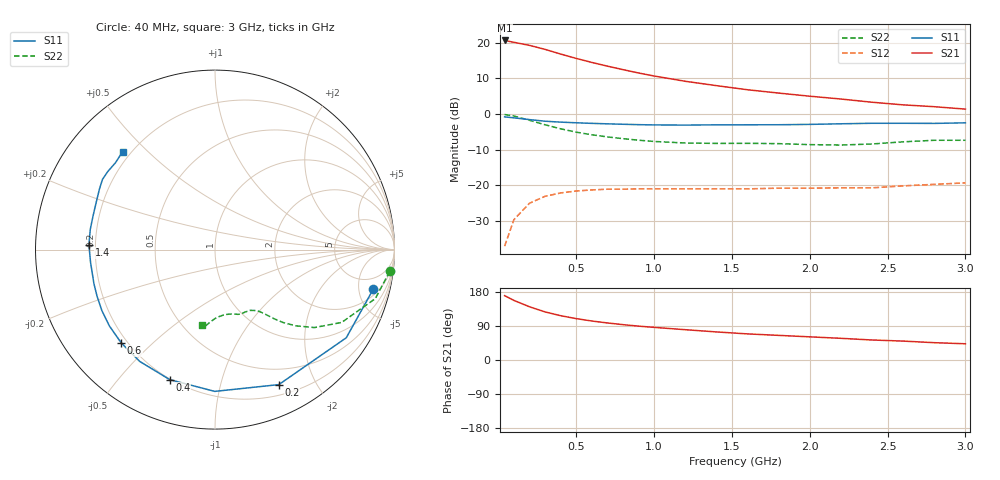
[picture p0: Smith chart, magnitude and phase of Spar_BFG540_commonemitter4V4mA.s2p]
! Filename:  BFG540A.S2P  Version:  3.0
! NXP part #: BFG540  Date: Feb 1992
! Bias condition: Vce=4V, Ic=4mA
! IN LINE PINNING: same data as with cross emitter pinning.
#  MHz  S  MA  R  50
! Freq  S11  S21  S12  S22  !GUM [dB]
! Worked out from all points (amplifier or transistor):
!   21 points, 40 MHz to 3 GHz, reference 50 ohm
!   highest |S21| = 20.6 dB at 40 MHz (marker M1)
!   |S21| within 3 dB of that: start of sweep to 337.9 MHz
!   unconditionally stable (mu >= 1): 1.751 GHz to end of sweep
!   at 300 MHz: K = 0.17, MSG = 20.6 dB, |S12| = -23.1 dB
!   at 1 GHz: K = 0.59, MSG = 15.8 dB, |S12| = -21.0 dB
!   at 3 GHz: K = 1.33, MAG = 6.9 dB, |S12| = -19.3 dB
!   S11 on the Smith chart (normalised r, x): 40 MHz: 2.79, -7.06; 200 MHz: 0.31, -1.53; 400 MHz: 0.20, -0.69; 600 MHz: 0.18, -0.40; 1.4 GHz: 0.17, +0.02; 3 GHz: 0.17, +0.42
40  0.909 -14.0  10.71 169.8  0.014 82.2  0.981 -7.1
100  0.881 -33.9  10.08 157.2  0.033 70.3  0.934 -17.0
200  0.832 -64.7  9.138 140.4  0.056 55.2  0.814 -29.9
300  0.79 -90.1  8.025 126.9  0.07 44.9  0.704 -38.1
400  0.767 -109.2  6.901 116.9  0.078 38.0  0.618 -43.4
500  0.751 -123.9  5.996 109.2  0.083 33.6  0.555 -47.0
600  0.737 -135.2  5.269 102.9  0.086 30.7  0.51 -49.3
700  0.726 -144.2  4.673 97.8  0.088 28.5  0.476 -51.0
800  0.716 -151.7  4.177 93.3  0.088 27.1  0.45 -52.5
900  0.707 -158.1  3.748 89.4  0.089 26.4  0.428 -54.0
1000  0.701 -164.1  3.4 86.1  0.089 26.3  0.411 -55.7
1200  0.697 -174.2  2.867 80.0  0.089 26.6  0.391 -60.0
1400  0.703 177.8  2.492 74.1  0.089 27.0  0.386 -64.4
1600  0.704 170.9  2.181 68.9  0.089 30.0  0.387 -67.6
1800  0.705 164.4  1.959 65.0  0.091 32.1  0.383 -70.4
2000  0.713 157.9  1.771 61.1  0.091 35.5  0.371 -74.9
2200  0.727 152.3  1.617 57.2  0.092 38.6  0.366 -81.6
2400  0.739 148.0  1.458 52.8  0.092 42.6  0.379 -88.8
2600  0.739 143.9  1.339 49.9  0.098 45.9  0.406 -94.1
2800  0.736 138.9  1.262 45.7  0.103 47.8  0.427 -96.9
3000  0.75 133.3  1.168 42.8  0.108 52.2  0.427 -99.8
